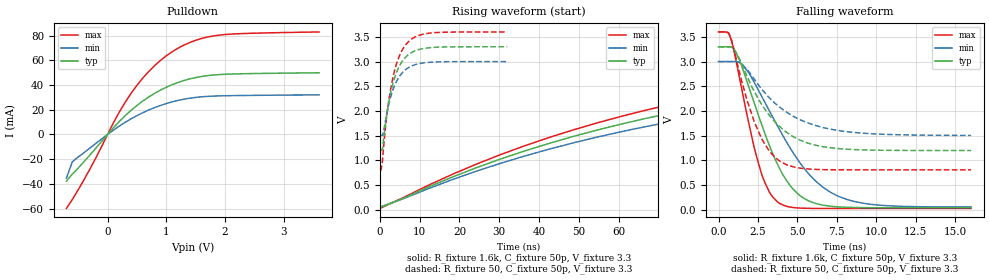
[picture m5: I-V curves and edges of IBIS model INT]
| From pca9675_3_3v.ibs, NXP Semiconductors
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[Model]   INT
Model_type Open_drain
Vref=3.3
Vmeas=1.65
Rref=500
Cref=50p
C_comp   5.2p   5p   5.4p
[Temperature Range] 27   85   -40
[Voltage Range]   3.3   3   3.6
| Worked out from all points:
|   slope of the pulldown table from 0 to 0.495 V, typ, clamps not added: 21.3 ohm
|   falling waveform, R_fixture 1.6k, C_fixture 50p, V_fixture 3.3: 20-80 % time 2.36ns typ, 3.42ns min, 1.52ns max; typ from 3.3 V to 0.037 V
|   falling waveform, R_fixture 50, C_fixture 50p, V_fixture 3.3: 20-80 % time 2.54ns typ, 3.17ns min, 1.74ns max; typ from 3.3 V to 1.2 V
|   rising waveform, R_fixture 1.6k, C_fixture 50p, V_fixture 3.3: 20-80 % time 112ns typ, 113ns min, 112ns max; typ from 0.037 V to 3.3 V
|   rising waveform, R_fixture 50, C_fixture 50p, V_fixture 3.3: 20-80 % time 3.52ns typ, 3.52ns min, 3.51ns max; typ from 1.2 V to 3.3 V
[Pulldown]
-700mV    -37.76mA   -35.32mA   -59.97mA
-600mV    -32.14mA   -22.14mA   -52.74mA
-300mV    -16.65mA   -11.05mA   -27.99mA
100mV     5.453mA    3.495mA    9.476mA
300mV     15.19mA    9.813mA    26.06mA
600mV     27.02mA    17.6mA     45.64mA
800mV     33.23mA    21.72mA    55.68mA
1V        38.22mA    25.02mA    63.67mA
1.4V      44.97mA    29.32mA    74.46mA
1.8V      48.09mA    31.03mA    79.74mA
2.3V      49.12mA    31.53mA    81.67mA
3.6V      49.91mA    32.03mA    82.97mA
[Falling Waveform]
R_fixture=1.6k
C_fixture=50p
V_fixture=3.3
V_fixture_min=3
V_fixture_max=3.6
0s        3.3V       3V         3.6V
646.5ps   3.3V       3V         3.577V
1.131ns   3.163V     2.999V     2.987V
2.263ns   2.162V     2.578V     1.254V
2.747ns   1.712V     2.289V     700.3mV
3.232ns   1.293V     1.995V     347.3mV
3.879ns   828.2mV    1.614V     122.9mV
5.495ns   213.5mV    809.4mV    26.97mV
7.758ns   52.15mV    248.7mV    22.92mV
16ns      36.62mV    52.66mV    22.88mV
[Falling Waveform]
R_fixture=50
C_fixture=50p
V_fixture=3.3
V_fixture_min=3
V_fixture_max=3.6
0s        3.3V       3V         3.6V
646.5ps   3.3V       3V         3.578V
969.7ps   3.259V     3V         3.261V
1.455ns   2.962V     2.957V     2.624V
2.263ns   2.398V     2.643V     1.785V
2.747ns   2.128V     2.437V     1.43V
4.202ns   1.593V     1.997V     926.1mV
5.657ns   1.348V     1.756V     824.1mV
8.081ns   1.225V     1.581V     805.8mV
16ns      1.197V     1.503V     805mV
[Rising Waveform]
R_fixture=1.6k
C_fixture=50p
V_fixture=3.3
V_fixture_min=3
V_fixture_max=3.6
0s        36.62mV    51.97mV    22.88mV
30.3ns    1.024V     937.3mV    1.114V
48.48ns   1.48V      1.35V      1.613V
66.67ns   1.845V     1.68V      2.012V
84.85ns   2.137V     1.944V     2.331V
109.1ns   2.437V     2.216V     2.659V
163.6ns   2.859V     2.6V       3.12V
224.2ns   3.091V     2.81V      3.373V
303ns     3.221V     2.928V     3.514V
600ns     3.298V     2.998V     3.598V
[Rising Waveform]
R_fixture=50
C_fixture=50p
V_fixture=3.3
V_fixture_min=3
V_fixture_max=3.6
0s        1.197V     1.502V     805mV
323.2ps   1.197V     1.502V     805mV
646.5ps   1.233V     1.502V     987.4mV
1.293ns   1.667V     1.748V     1.569V
1.939ns   2.032V     2.025V     2.024V
3.232ns   2.539V     2.415V     2.659V
4.848ns   2.898V     2.691V     3.103V
6.788ns   3.113V     2.857V     3.37V
12.61ns   3.281V     2.986V     3.577V
32ns      3.3V       3V         3.6V
[Ramp]
R_load=1.6k
dV/dt_r   1.958E+0/1.851E-9   1.946E+0/2.033E-9   1.967E+0/1.628E-9
dV/dt_f   1.958E+0/1.637E-10   1.946E+0/2.065E-10   1.967E+0/7.359E-11
|[End   INT
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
